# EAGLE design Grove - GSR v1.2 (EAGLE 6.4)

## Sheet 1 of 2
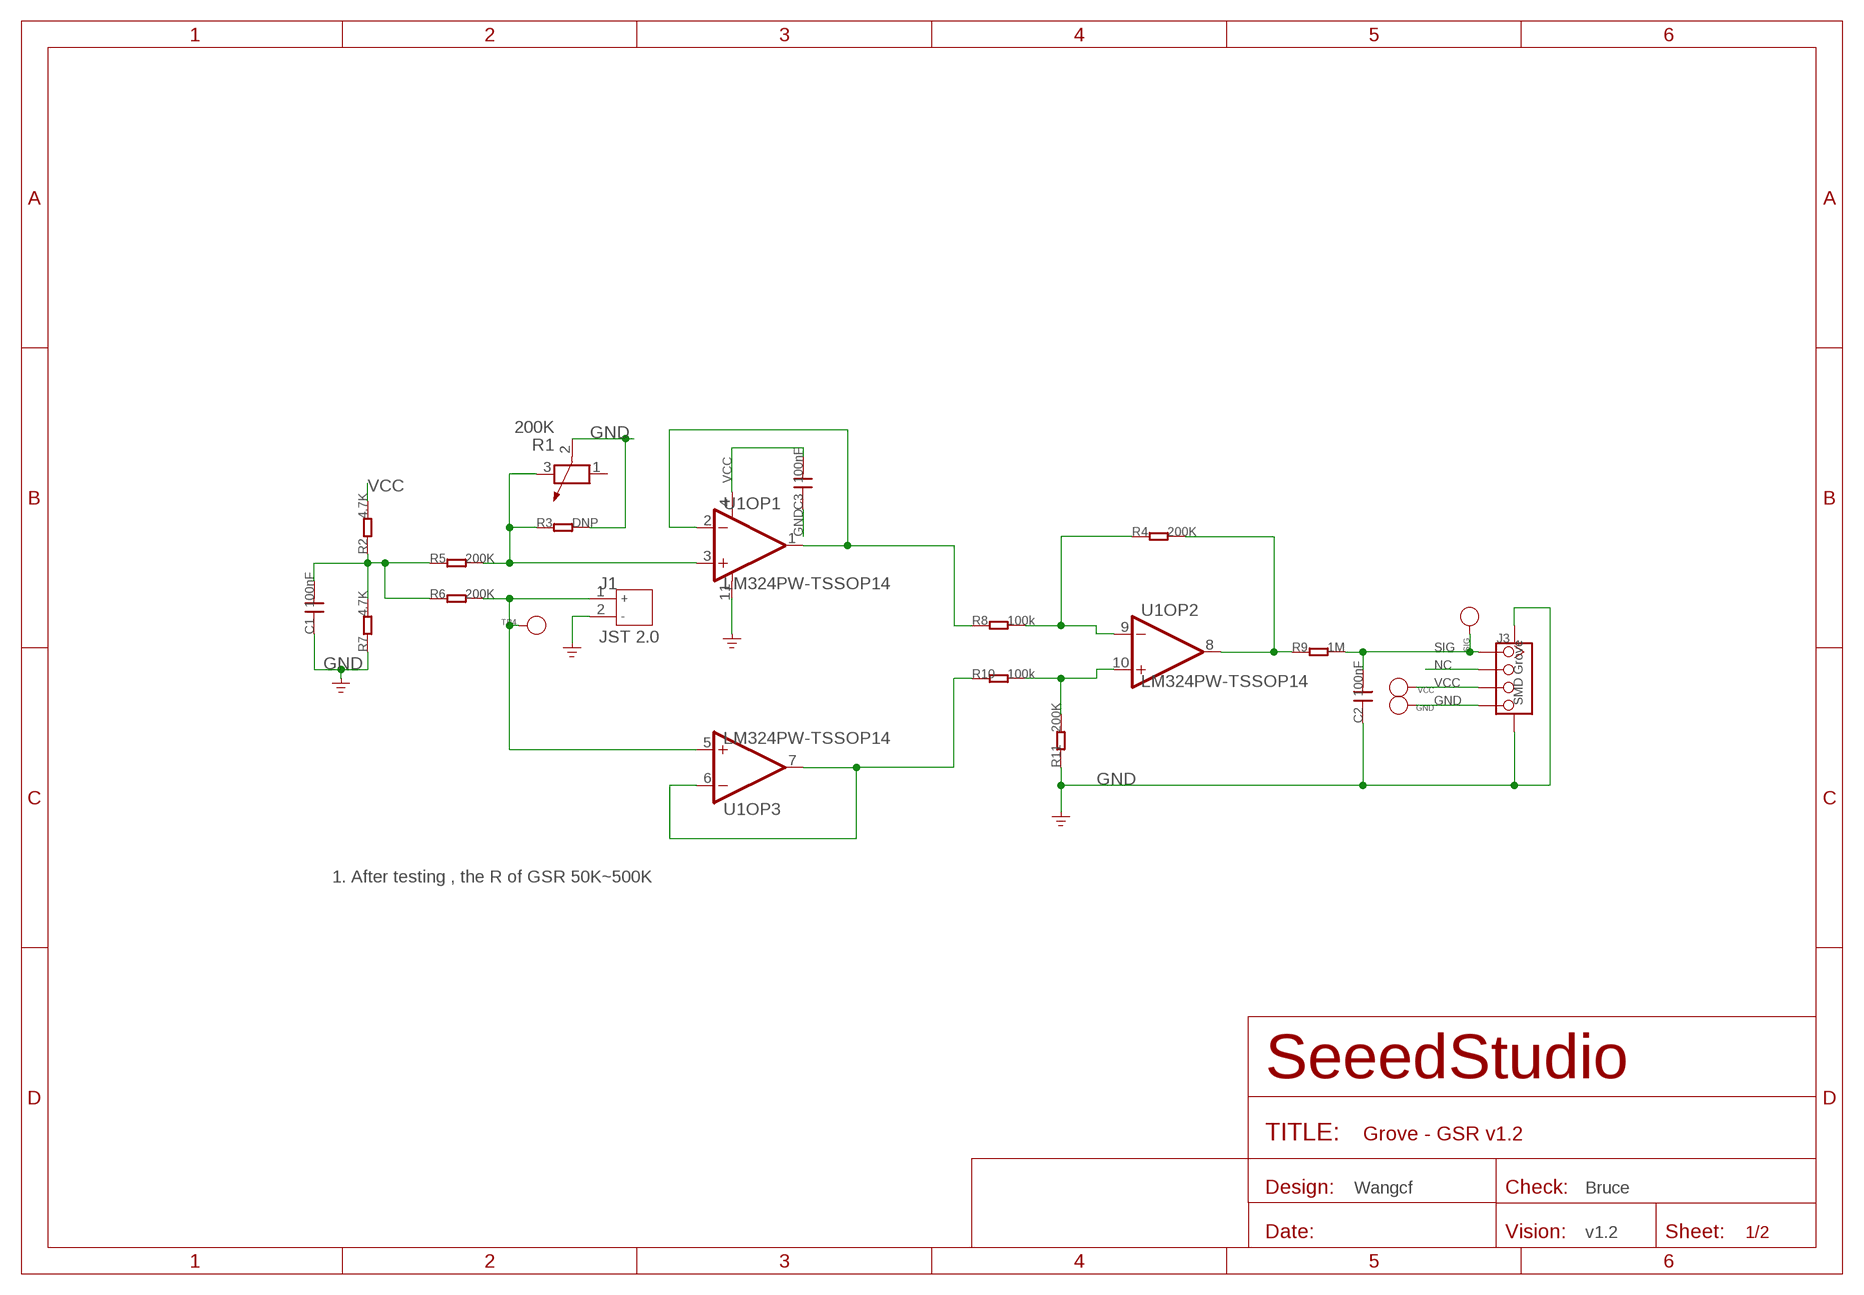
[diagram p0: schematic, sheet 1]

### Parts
C1  100nF  C-0603  [0603]
C2  100nF  C-0603  [0603]
C3  100nF  C-0603  [0603]
GND  PAD-TEST-POINT'4545'  [TP_4545]
J1  JST 2.0  JACK-JST-2P-PW'2.0'  [JST-2.0]
J3  SMD Grove  TWIG-4P-2.0-SMD-FEMALE-REINFORCE'DD'  [4P-SMD-2.0]
R1  200K  R-POTENTIOMETER-SMD  [3P-SMD-RECT-3.3X3.6]
R2  4.7K  R-0603  [0603]
R3  DNP  R-0603  [0603]
R4  200K  R-0603  [0603]
R5  200K  R-0603  [0603]
R6  200K  R-0603  [0603]
R7  4.7K  R-0603  [0603]
R8  100k  R-0603  [0603]
R9  1M  R-0603  [0603]
R10  100k  R-0603  [0603]
R11  200K  R-0603  [0603]
SIG  PAD-TEST-POINT'4545'  [TP_4545]
TP4  PAD-TEST-POINT'4545'  [TP_4545]
U1  LM324PW-TSSOP14  LMV324-TSSOP14  [TSSOP14]
VCC  PAD-TEST-POINT'4545'  [TP_4545]

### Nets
GND: C1.1 C2.1 C3.1 GND.T J1.2 J3.4 J3.SS1 J3.SS2 R1.2 R3.2 R7.1 R11.1 U1.11(OP1:V-)
IN: J1.1 R6.2 TP4.T U1.5(OP3:IN+)
N$1: R8.1 U1.1(OP1:OUT) U1.2(OP1:IN-)
N$2: R10.1 U1.6(OP3:IN-) U1.7(OP3:OUT)
N$3: R4.1 R8.2 U1.9(OP2:IN-)
N$4: R4.2 R9.1 U1.8(OP2:OUT)
N$5: R10.2 R11.2 U1.10(OP2:IN+)
N$6: C1.2 R2.1 R5.1 R6.1 R7.2
N$8: R1.3 R3.1 R5.2 U1.3(OP1:IN+)
NC: J3.2
SIG: C2.2 J3.1 R9.2 SIG.T
VCC: C3.2 J3.3 R2.2 U1.4(OP1:V+) VCC.T
Unconnected: R1.1 U1.12(OP4:IN+) U1.13(OP4:IN-) U1.14(OP4:OUT)

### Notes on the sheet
- 1. After testing , the R of GSR 50K~500K
- Wangcf | Bruce
- v1.2

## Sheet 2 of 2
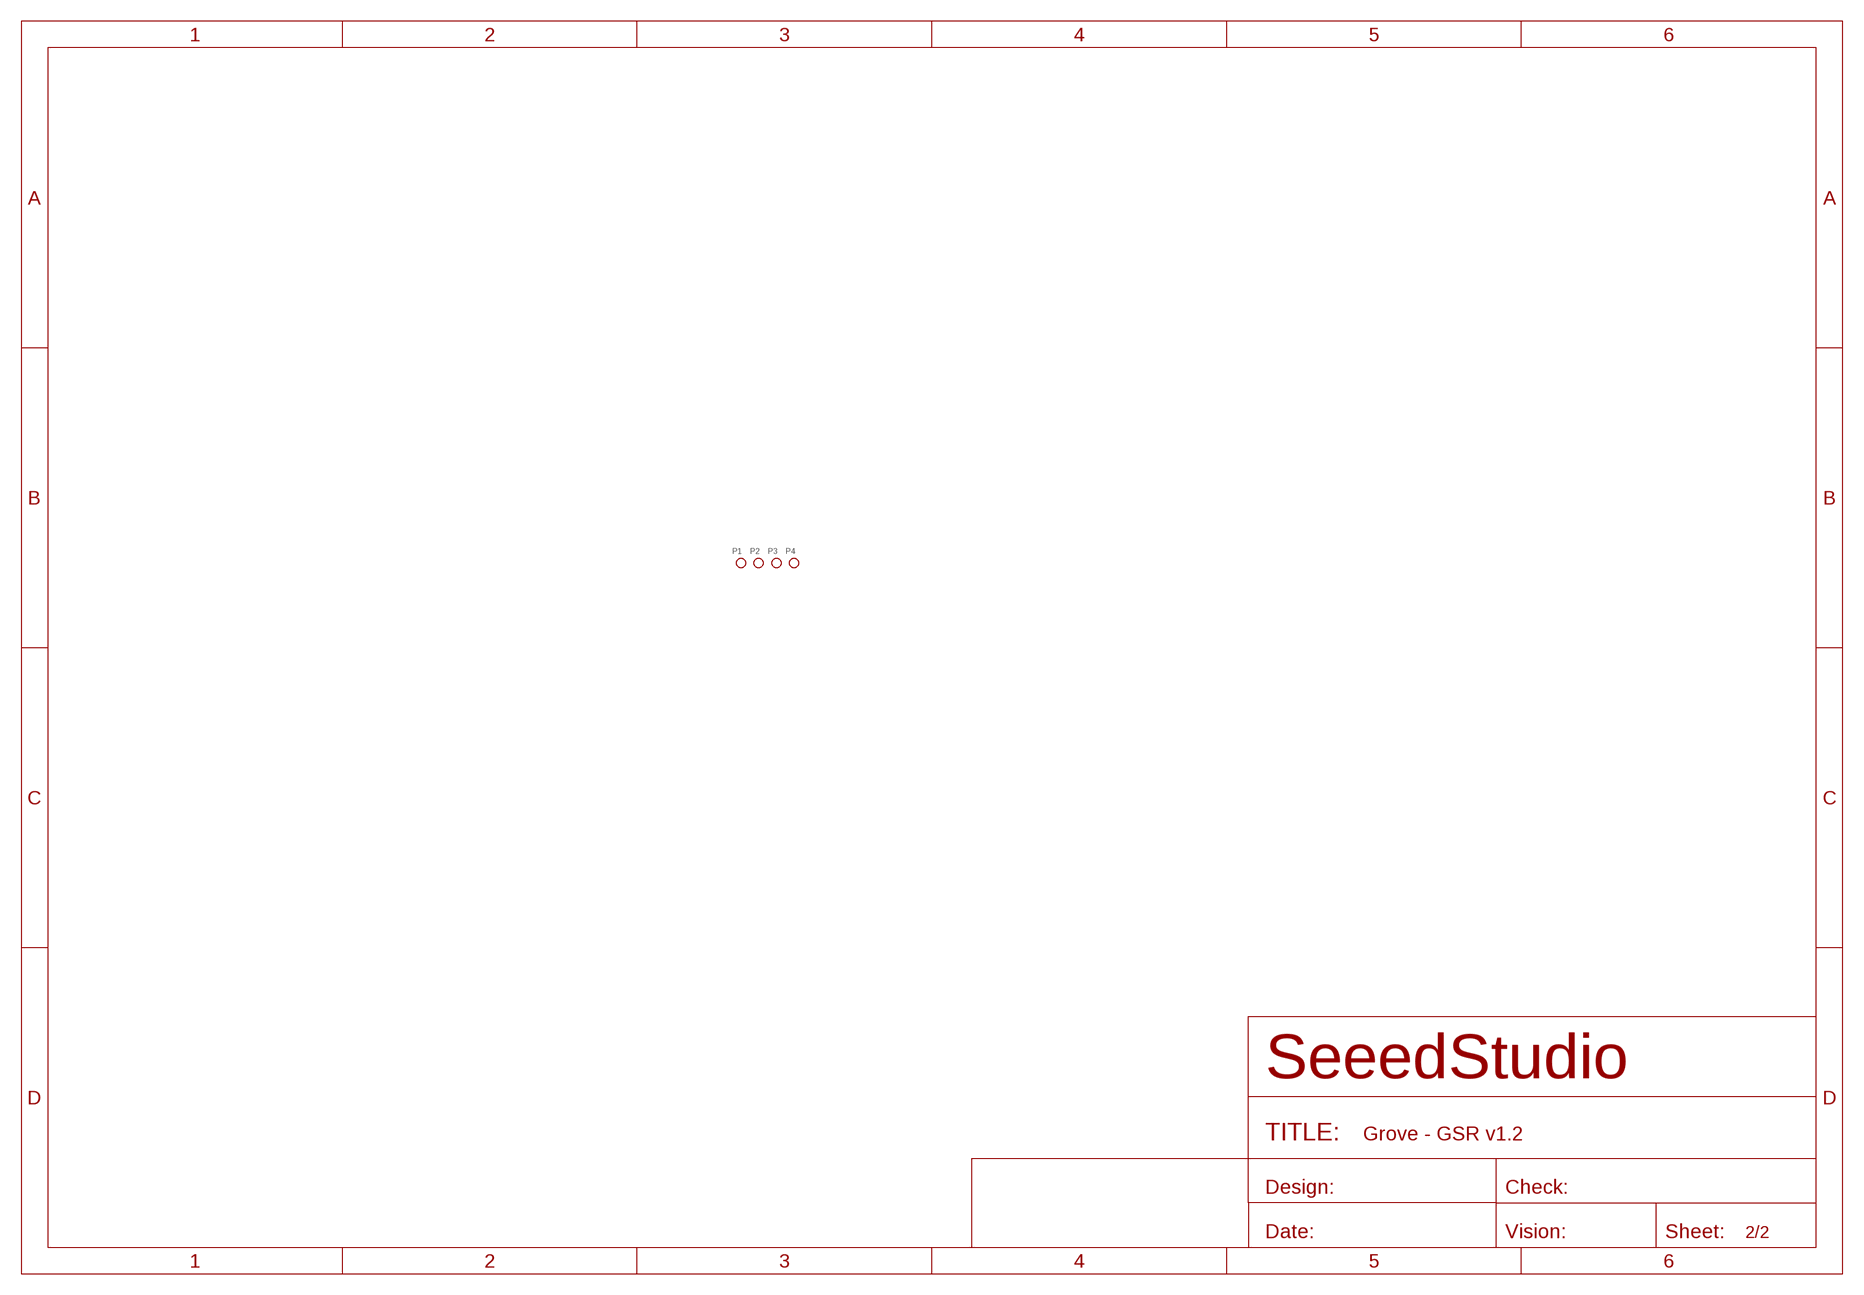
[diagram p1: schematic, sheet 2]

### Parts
P1  PAD-MARK  [ROUND-MARK-1.0]
P2  PAD-MARK  [ROUND-MARK-1.0]
P3  PAD-MARK  [ROUND-MARK-1.0]
P4  PAD-MARK  [ROUND-MARK-1.0]

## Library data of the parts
C1-C3 = Discreter:C*: Ceramic Capacitors
GND SIG TP4 VCC = Discrete:PAD-TEST-POINT; PARTNO: DNP
J1 = Connector:JACK-JST-2P-PW
J3 = Connector:TWIG-4P-2.0-SMD-FEMALE-REINFORCE
P1-P4 = Discrete:PAD-MARK; PARTNO: DNP
R1 = Discreter:R-POTENTIOMETER*: Potentiometer
R2-R11 = Discreter:R*
U1 = IC:LMV324: General purpose LOW Voltage, Rail-to-Rail Output Amplifiers http://www.fairchildsemi.com/ds/LM/LMV358.pdf

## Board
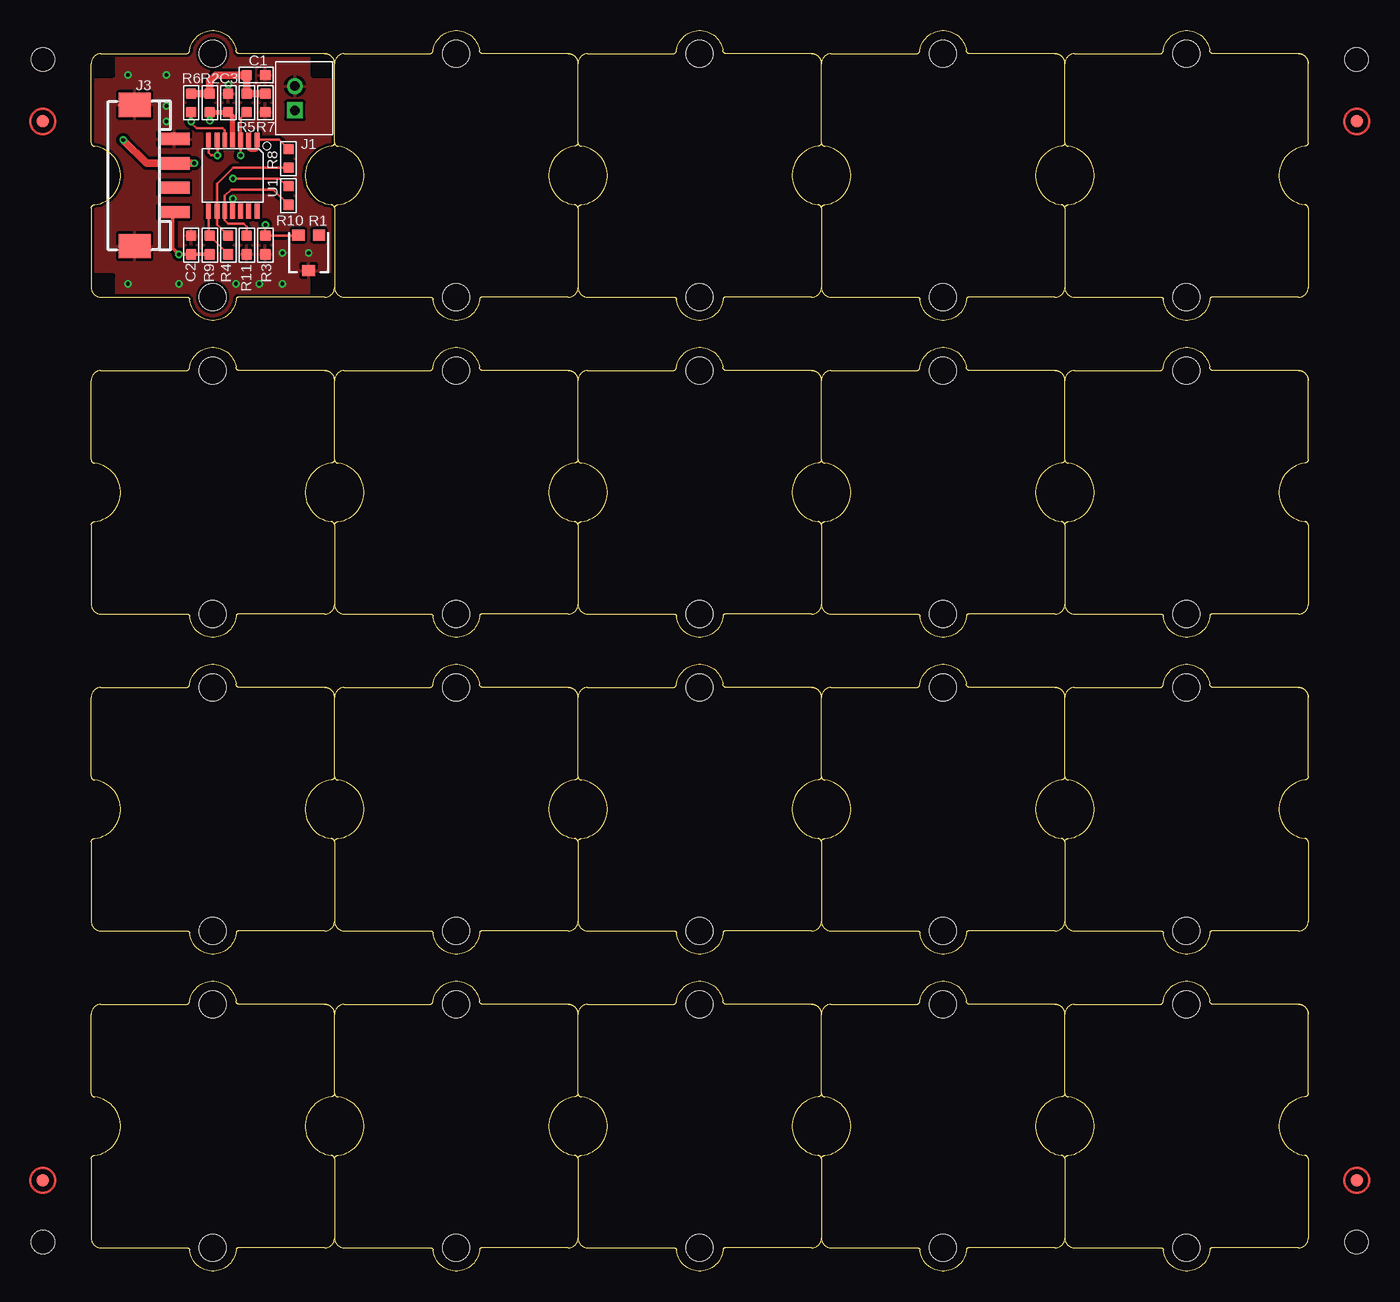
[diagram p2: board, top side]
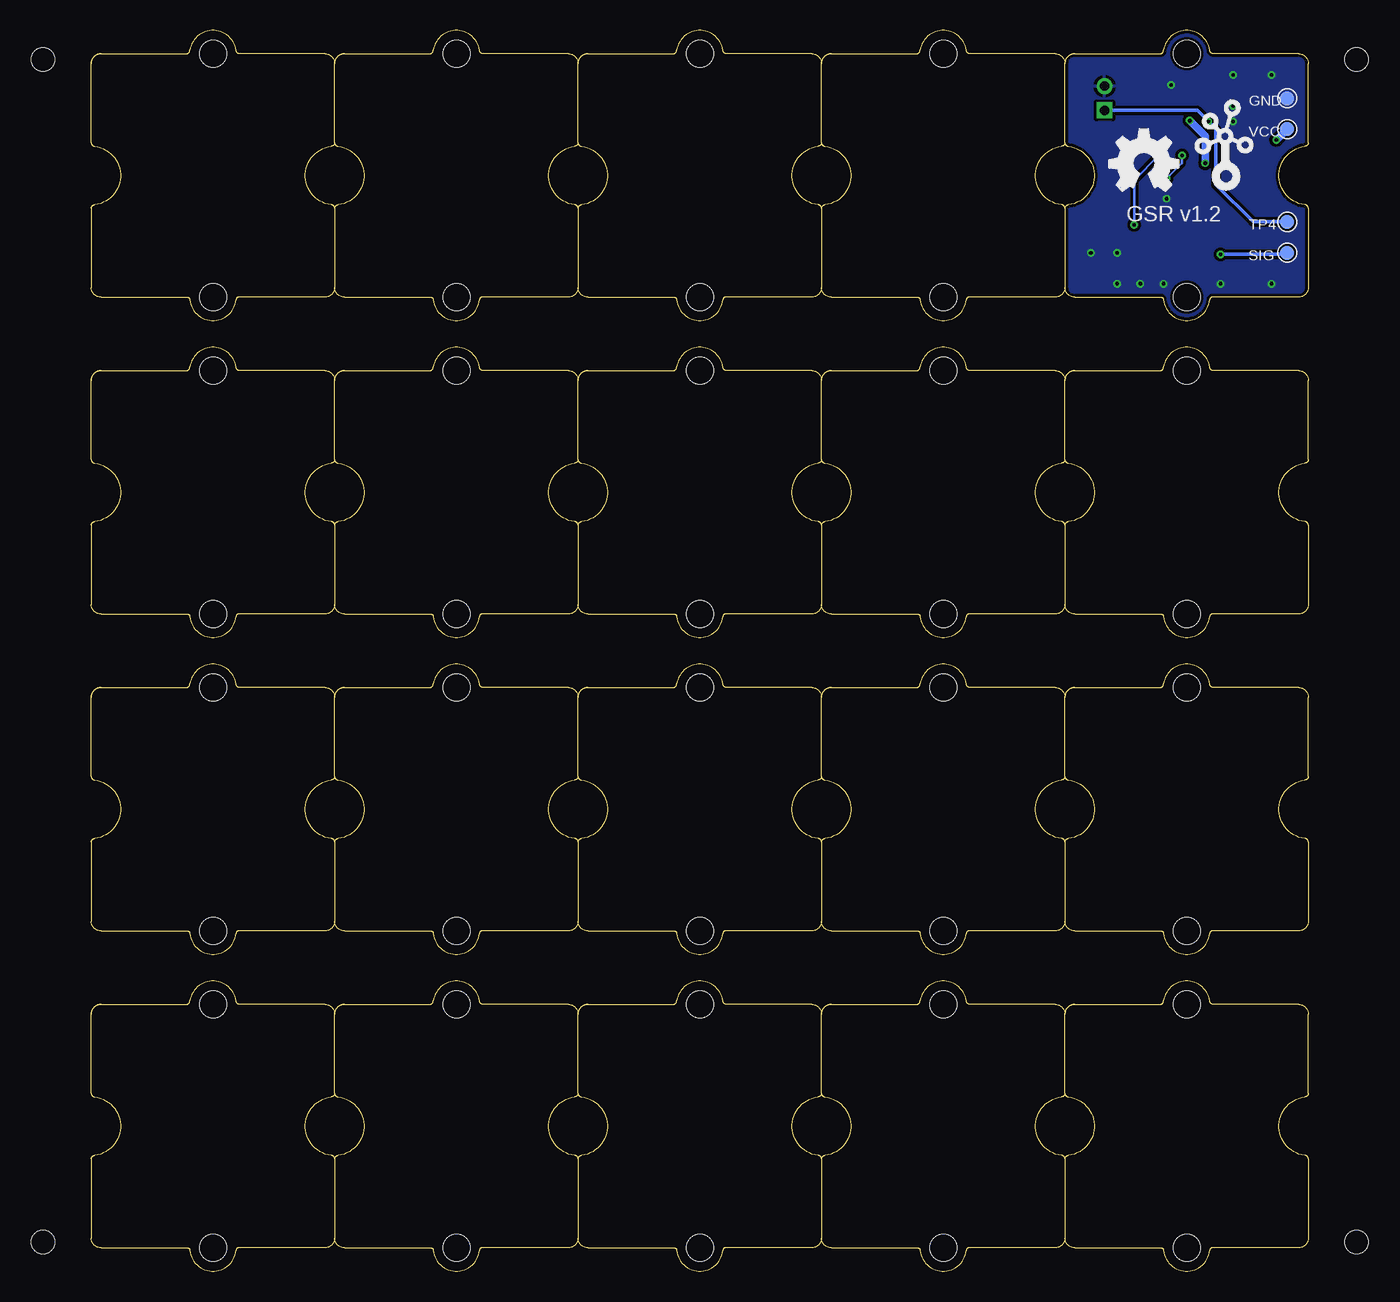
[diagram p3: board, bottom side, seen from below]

Size 100 x 101.93 mm. Coordinates in mm from the lower left corner, seen from the top.
Copper layers (1*16): Top 0.035mm / dielectric 1.5mm / Bottom 0.035mm
Design rules "SeeedStudio_rule_no_angle_090911 *": minimum track width 6mil, minimum drill 12mil, track to track 6mil, track to pad 6mil, pad to pad 6mil, via to via 6mil, smd to smd 0mil, copper to edge 10mil, drill to drill 10mil, minimum pad ring 10mil, minimum via ring 6mil, stop-mask expansion 2mil, vias tented up to drill 100mil, thermal gap 10mil
Holes 1.91 mm at -3.97,2.38 -3.97,99.54 103.98,99.54 103.98,2.38

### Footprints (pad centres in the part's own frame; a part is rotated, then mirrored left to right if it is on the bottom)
0603 = smd 0.889 x 0.889: 1 -0.762,0; 2 0.762,0
TP_4545 = smd 1.143 x 1.143: T 0,0
JST-2.0 = drill 0.8 pad 1.3 square: 1 -1,0.75 | drill 0.8 pad 1.3: 2 1,0.75
4P-SMD-2.0 = smd 1 x 2.54: 1 -3,0; 2 -1,0; 3 1,0; 4 3,0 | smd 2 x 2.6: SS1 -5.8,3.25; SS2 5.8,3.25
ROUND-MARK-1.0 = smd 1.016 x 1.016: P$1 0,0
3P-SMD-RECT-3.3X3.6 = smd 1 x 0.9: 1 -0.85,-1.45; 3 0.85,-1.45 | smd 1.1 x 0.9: 2 0,1.45
TSSOP14 = smd 0.4 x 1.2: 1 -2,-2.925; 2 -1.3,-2.925; 3 -0.65,-2.925; 4 0,-2.925; 5 0.65,-2.925; 6 1.3,-2.925; 7 2,-2.925; 8 2,2.925; 9 1.3,2.925; 10 0.65,2.925; 11 0,2.925; 12 -0.65,2.925; 13 -1.3,2.925; 14 -2,2.925
1U-DIM-W/-DRILL = hole 2.2: 0,-10; 0,10

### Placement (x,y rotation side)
C1  13.56,98.27 180 top
C2  8.22,84.3 270 top
C3  11.27,95.98 270 top
GND  1.74,96.36 0 bottom
J1  17.49,96.36 90 top
J3  6.83,90.01 90 top
P1  not placed on the board
P2  not placed on the board
P3  not placed on the board
P4  not placed on the board
R1  17.87,83.66 180 top
R2  9.75,95.98 270 top
R3  14.32,84.3 270 top
R4  11.27,84.3 270 top
R5  12.79,95.98 270 top
R6  8.22,95.98 270 top
R7  14.32,95.98 90 top
R8  16.22,91.41 270 top
R9  9.75,84.3 270 top
R10  16.22,88.36 270 top
R11  12.79,84.3 90 top
SIG  1.74,83.66 0 bottom
TP4  1.74,86.2 0 bottom
U1  11.64,90.01 180 top
U$7  [TWIGLOGO]  6.83,89.76 0 bottom
U$8  [OSHW_FILLX200_NOTEXT]  16.35,88.74 0 bottom
U$9  [1U-DIM-W/-DRILL]  10,90.01 0 top
U$10  [1U-DIM-W/-DRILL]  10,90.01 0 top
U$11  [1U-DIM-W/-DRILL]  30,90.01 0 top
U$12  [1U-DIM-W/-DRILL]  50,90.01 0 top
U$13  [1U-DIM-W/-DRILL]  70,90.01 0 top
U$14  [1U-DIM-W/-DRILL]  90,90.01 0 top
U$15  [1U-DIM-W/-DRILL]  30,63.98 0 top
U$16  [1U-DIM-W/-DRILL]  50,63.98 0 top
U$17  [1U-DIM-W/-DRILL]  70,63.98 0 top
U$18  [1U-DIM-W/-DRILL]  90,63.98 0 top
U$19  [1U-DIM-W/-DRILL]  10,63.98 0 top
U$20  [1U-DIM-W/-DRILL]  30,37.94 0 top
U$21  [1U-DIM-W/-DRILL]  50,37.94 0 top
U$22  [1U-DIM-W/-DRILL]  70,37.94 0 top
U$23  [1U-DIM-W/-DRILL]  90,37.94 0 top
U$24  [1U-DIM-W/-DRILL]  10,37.94 0 top
U$25  [1U-DIM-W/-DRILL]  30,11.91 0 top
U$26  [1U-DIM-W/-DRILL]  50,11.91 0 top
U$27  [1U-DIM-W/-DRILL]  70,11.91 0 top
U$28  [1U-DIM-W/-DRILL]  90,11.91 0 top
U$29  [1U-DIM-W/-DRILL]  10,11.91 0 top
VCC  1.74,93.82 0 bottom

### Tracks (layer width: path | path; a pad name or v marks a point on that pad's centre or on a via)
GND  (via drill 0.3 pad 0.51)
  other vias: 11.27,97.44 15.71,81.12 17.87,83.66 15.71,83.66 13.81,81.12 11.9,81.12 7.21,81.12 3.01,81.12 6.19,94.46 6.19,95.73 6.19,98.27 3.01,98.27 11.65,88.11
  pour Bottom (isolate 0.254): -0.16,102.08 20.29,102.08 20.29,77.95 -0.16,77.95
  pour Top (isolate 0.254): -0.16,102.08 20.29,102.08 20.29,77.95 -0.16,77.95
IN  (via drill 0.3 pad 0.51)
  Top 0.203: U1.5 10.99,93.72 10.83,93.89 8.67,93.89 8.22,94.33 v8.22,94.46 | 8.22,95.09 R6.2
  Top 0.305: v8.22,94.46 8.22,95.09
  Bottom 0.305: TP4.T 4.54,86.2 7.59,89.25 7.59,93.82 v8.22,94.46 9.05,95.28 9.1,95.33 9.13,95.36 J1.1
N$1
  Top 0.203: U1.2 12.94,92.15 13.05,92.05 13.54,92.05 13.64,92.15 U1.1 15.46,92.94 R8.1
N$2  (via drill 0.3 pad 0.51)
  Top 0.203: R10.1 16.1,89.12 15.46,89.76 v11.65,89.76 | U1.6 10.38,92.9 v10.38,91.66 9.87,91.66 9.64,91.9 U1.7
  Bottom 0.203: v11.65,89.76 10.38,91.03 v10.38,91.66
N$3
  Top 0.203: R8.2 11.65,90.65 10.34,89.34 U1.9 10.34,85.99 R4.1
N$4
  Top 0.203: U1.8 9.64,85.16 R9.1 R4.2
N$5
  Top 0.203: R10.2 14.95,88.87 11.52,88.87 10.99,88.34 U1.10 10.99,86.35 11.27,86.08 12.54,86.08 12.79,85.82 R11.2
N$6
  Top 0.61: R7.2 R5.1 C1.2 10.25,98.27 9.75,97.76 R2.1 R6.1
N$8  (via drill 0.3 pad 0.51)
  Top 0.203: R5.2 12.29,94.72 U1.3 v12.29,91.66 | R1.3 16.97,85.06 R3.1 v14.32,85.95
  Bottom 0.203: v14.32,85.95 14.32,89.63 v12.29,91.66
SIG  (via drill 0.3 pad 0.51)
  Top 0.203: 6.7,86.89 J3.1
  Top 0.305: 6.7,86.89 6.7,84.04 v7.21,83.54 C2.2 R9.2
  Bottom 0.305: v7.21,83.54 2.13,83.54 1.87,83.79 SIG.T
VCC  (via drill 0.3 pad 0.51)
  Top 0.406: U1.4 11.64,94.85 C3.2 R2.2 v9.75,94.52
  Top 0.61: v8.48,91.03 8.46,91.01 J3.3 4.55,91.01 v2.63,92.93
  Bottom 0.61: v8.48,91.03 8.48,93.25 v9.75,94.52 | v2.63,92.93 VCC.T

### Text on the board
bPlace: GSR v1.2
